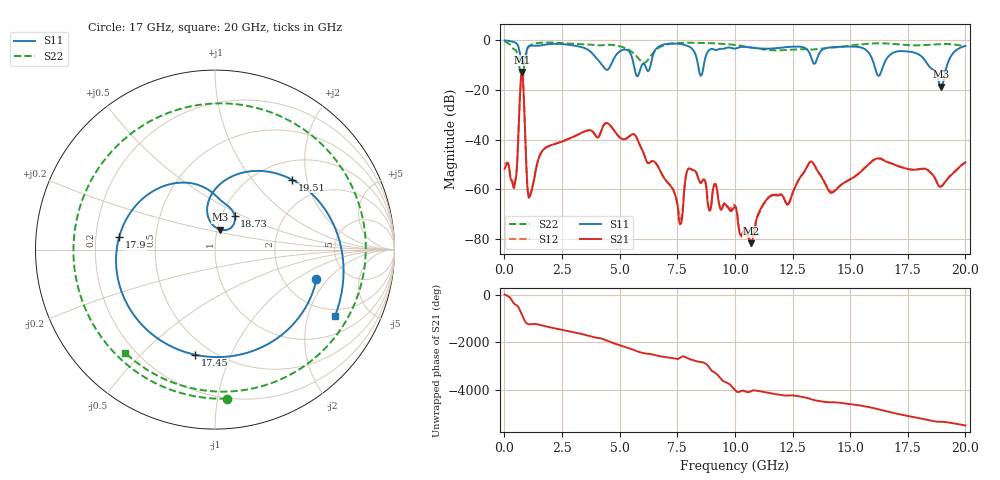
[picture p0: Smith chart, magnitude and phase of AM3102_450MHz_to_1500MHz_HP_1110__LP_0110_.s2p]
!Agilent Technologies,E8364B,MY43040894,A.07.50.67
!Agilent E8364B: A.07.50.67
!Date: Thursday, January 11, 2018 06:43:42
!Correction: S11(Full 2 Port(1,2))
!S21(Full 2 Port(1,2))
!S12(Full 2 Port(1,2))
!S22(Full 2 Port(1,2))
!S2P File: Measurements: S11, S21, S12, S22:
# Hz S  dB  R 50
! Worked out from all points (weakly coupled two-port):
!   1601 points, 10 MHz to 20 GHz, reference 50 ohm
!   highest |S21| = -12.83 dB at 759.6 MHz (marker M1); lowest = -81.7 dB at 10.7 GHz (marker M2)
!   lowest |S11| = -18.8 dB at 18.95 GHz (marker M3), VSWR 1.26, Z = 51.6 + j11.7 ohm
!   |S11| at or under -10 dB: 4.244 GHz to 4.617 GHz (373.8 MHz wide, 8.44 % of centre); 16.05 GHz to 16.45 GHz (401.2 MHz wide, 2.47 % of centre); 18.39 GHz to 19.21 GHz (822.5 MHz wide, 4.38 % of centre)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
!   |S22| runs from -14.9 to -0.5 dB; largest |S21 - S12| = 0.00097
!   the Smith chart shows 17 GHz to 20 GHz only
!   S11 on the Smith chart (normalised r, x): 17 GHz: 3.03, -1.52; 17.45 GHz: 0.41, -0.74; 17.9 GHz: 0.30, +0.06; 18.73 GHz: 1.15, +0.45; 19.51 GHz: 1.39, +1.63; 20 GHz: 1.68, -3.00
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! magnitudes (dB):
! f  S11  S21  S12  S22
! 10 MHz  -0.1  -51.8  -49.8  -0.5
! 459.8 MHz  -0.9  -57.5  -56.8  -3.8
! 759.6 MHz  -8.9  -12.8  -12.8  -14.8
! 1.097 GHz  -2.3  -63.0  -62.5  -2.2
! 1.684 GHz  -1.9  -44.1  -44.1  -1.0
! 3.346 GHz  -2.8  -37.3  -37.3  -1.6
! 5.77 GHz  -14.5  -39.8  -39.8  -6.8
! 6.682 GHz  -2.7  -51.1  -51.0  -3.2
! 7.644 GHz  -1.5  -73.9  -72.0  -1.1
! 8.043 GHz  -2.7  -51.7  -51.6  -1.0
! 10.01 GHz  -3.4  -66.9  -66.5  -1.9
! 10.7 GHz  -2.9  -81.7  -82.9  -2.9
! 13.34 GHz  -7.8  -48.9  -48.8  -3.8
! 14.2 GHz  -2.8  -61.3  -60.9  -3.0
! 16.68 GHz  -6.4  -49.2  -49.2  -1.4
! 17 GHz  -4.6  -50.3  -50.3  -1.6
! 17.45 GHz  -4.5  -51.7  -51.6  -1.9
! 17.9 GHz  -5.4  -52.0  -52.1  -2.1
! 18.73 GHz  -13.3  -56.5  -56.4  -1.6
! 18.95 GHz  -18.8  -58.8  -58.8  -1.5
! 19.51 GHz  -4.7  -53.1  -53.0  -1.8
! 20 GHz  -2.3  -49.1  -49.4  -2.4
